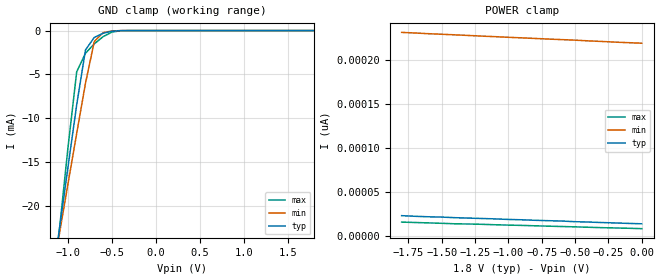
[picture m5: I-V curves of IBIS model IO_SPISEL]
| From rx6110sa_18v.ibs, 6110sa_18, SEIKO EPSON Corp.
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[Model]   IO_SPISEL
Model_type Input
Enable Active-High
Polarity Non-Inverting
Vinh=1.26
Vinl=0.54
C_comp   2.5p   2p   3p
[Temperature Range] 25   85   -40
[Voltage Range]   1.8   1.6   2.0
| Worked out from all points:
|   GND clamp passes 1 mA (typ) near -0.72 V on its own axis
[GND Clamp]
-1.8V     -75.19mA   -65.43mA   -91.91mA
-1.1V     -22.89mA   -23.37mA   -23.06mA
-1V       -15.64mA   -17.52mA   -13.43mA
-900mV    -8.46mA    -11.72mA   -4.701mA
-800mV    -2.2mA     -5.996mA   -2.58mA
-700mV    -777.8uA   -1.246mA   -1.512mA
-600mV    -308.2uA   -237.4uA   -691.5uA
-500mV    -74.58uA   -42.13uA   -176.4uA
-400mV    -7.855uA   -4.907uA   -14.74uA
1.8V      13.7pA     219.9pA    7.39pA
[POWER Clamp]
-1.8V     22.96pA    230.9pA    15.69pA
-1.7V     22.28pA    230.2pA    15.23pA
-1.6V     21.71pA    229.4pA    14.78pA
-1.5V     21.37pA    228.8pA    14.32pA
-1.4V     20.69pA    228.1pA    13.76pA
-1.2V     19.78pA    226.7pA    13.19pA
-1.1V     19.33pA    226.1pA    12.68pA
-1V       18.7pA     225.3pA    12.28pA
-600mV    16.88pA    222.7pA    10.69pA
-500mV    16.14pA    222.1pA    10.29pA
-200mV    14.72pA    219.9pA    9.038pA
0V        13.76pA    218.6pA    8.242pA
